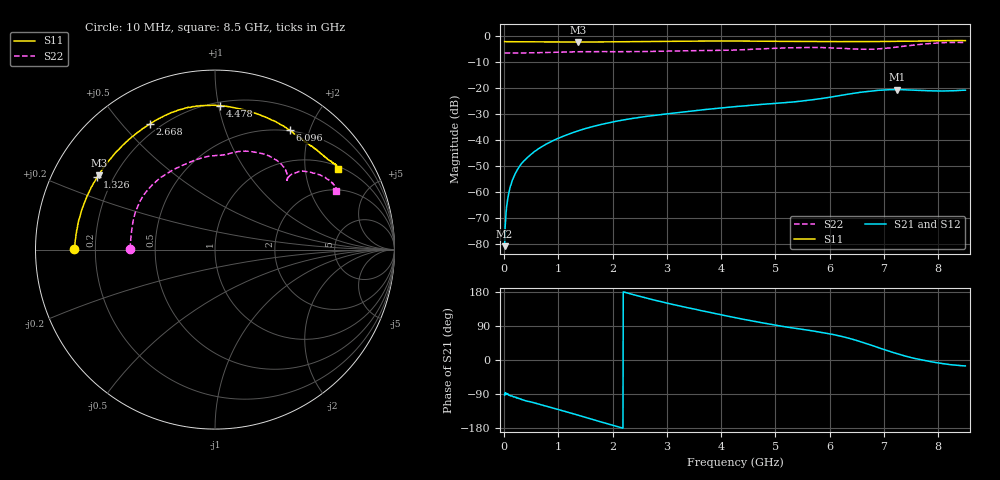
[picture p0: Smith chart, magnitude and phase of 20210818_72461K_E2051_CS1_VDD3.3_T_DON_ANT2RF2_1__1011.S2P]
!Agilent Technologies,E5071C,MY46417908,A.11.23
!Date: Wed Aug 18 14:27:52 2021
!Data & Calibration Information:
!Freq	S11:SOLT2(ON)	S21:SOLT2(ON)	S12:SOLT2(ON)	S22:SOLT2(ON)
!PortZ  Port1:50+j0  Port2:50+j0
!Above PortZ is port z conversion or system Z0 setting when saving the data.
!When reading, reference impedance value at option line is always used.
# Hz S dB R 50
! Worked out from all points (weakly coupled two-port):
!   1601 points, 10 MHz to 8.5 GHz, reference 50 ohm
!   highest |S21| = -20.59 dB at 7.248 GHz (marker M1); lowest = -80.9 dB at 10 MHz (marker M2)
!   lowest |S11| = -2.3 dB at 1.368 GHz (marker M3), VSWR 7.68, Z = 7.06 + j14.4 ohm
!   |S11| at or under -10 dB: nowhere
!   |S22| runs from -6.5 to -2.4 dB; largest |S21 - S12| = 0.00048
!   S11 on the Smith chart (normalised r, x): 10 MHz: 0.12, +0.00; 1.326 GHz: 0.14, +0.28; 2.668 GHz: 0.16, +0.60; 4.478 GHz: 0.22, +1.01; 6.096 GHz: 0.49, +1.70; 8.5 GHz: 1.11, +3.00
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1e7  -2.11 179.7  -80.95 -92.7  -79.56 -86.5  -6.47 179.6
6.30625e7  -2.14 178.5  -63.16 -90.5  -63.21 -89.4  -6.49 178.3
1.055125e8  -2.15 177.6  -58.70 -93.6  -58.61 -93.1  -6.50 177.1
1.851062e8  -2.17 175.7  -53.93 -97.1  -53.91 -97.3  -6.51 174.9
3.018438e8  -2.19 173.0  -49.65 -102.6  -49.64 -103.2  -6.51 172.1
5.194e8  -2.19 168.1  -45.17 -111.2  -45.16 -111.4  -6.44 166.6
7.10425e8  -2.22 163.4  -42.40 -119.3  -42.41 -119.3  -6.34 161.4
1.32595e9  -2.27 148.4  -36.78 -144.0  -36.79 -144.1  -6.03 143.2
1.3684e9  -2.28 147.4  -36.49 -145.8  -36.49 -145.8  -6.02 142.0
1.426769e9  -2.26 145.8  -36.07 -148.3  -36.10 -148.1  -6.01 140.2
2.036988e9  -2.20 130.8  -32.93 -173.7  -32.94 -173.7  -6.01 122.4
2.668431e9  -2.07 117.3  -30.83 161.8  -30.82 161.8  -5.93 107.0
2.843538e9  -2.02 114.2  -30.37 155.5  -30.37 155.5  -5.85 103.3
4.255e9  -1.89 91.7  -27.19 111.9  -27.19 111.9  -5.36 81.8
4.477862e9  -1.92 87.9  -26.79 105.7  -26.79 105.8  -5.17 79.0
5.671769e9  -2.06 64.9  -24.55 77.1  -24.57 77.2  -4.38 55.7
6.096269e9  -2.09 58.0  -23.25 66.2  -23.28 66.2  -4.57 48.1
6.610975e9  -2.13 51.0  -21.53 46.3  -21.54 46.1  -5.07 43.8
7.088538e9  -2.04 46.1  -20.66 23.5  -20.68 23.4  -4.56 44.7
7.247725e9  -2.00 44.6  -20.59 16.2  -20.60 16.2  -4.19 43.7
8.048969e9  -1.77 36.2  -21.17 -9.0  -21.15 -9.0  -2.58 31.3
8.5e9  -1.74 33.0  -20.83 -15.6  -20.83 -15.9  -2.51 25.8
